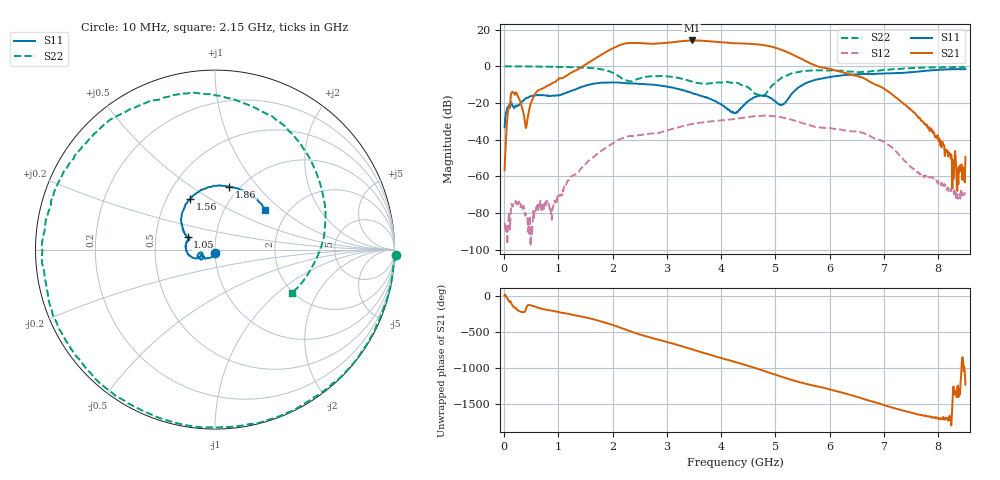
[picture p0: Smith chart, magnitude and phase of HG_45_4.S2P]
!Agilent Technologies,E5071C,MY46523237,B.13.01
!Date: Tue Sep 12 16:48:18 2023
!Data & Calibration Information:
!Freq	S11:SOLT2(ON)	S21:SOLT2(ON)	S12:SOLT2(ON)	S22:SOLT2(ON)
!PortZ  Port1:50+j0  Port2:50+j0
!Above PortZ is port z conversion or system Z0 setting when saving the data.
!When reading, reference impedance value at option line is always used.
# Hz S dB R 50
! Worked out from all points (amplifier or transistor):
!   850 points, 10 MHz to 8.5 GHz, reference 50 ohm
!   highest |S21| = 14.1 dB at 3.46 GHz (marker M1)
!   |S21| within 3 dB of that: 2.092 GHz to 4.878 GHz (2.786 GHz wide, 79.9 % of centre)
!   unconditionally stable (mu >= 1): 23.91 MHz to end of sweep
!   at 1.42 GHz: K = 40.33, MAG = 8.5 dB, |S12| = -55.8 dB
!   at 4.26 GHz: K = 2.85, MAG = 13.2 dB, |S12| = -28.6 dB
!   at 8.5 GHz: K = 14264.41, MAG = -34.9 dB, |S12| = -68.8 dB
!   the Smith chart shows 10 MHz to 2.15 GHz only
!   S11 on the Smith chart (normalised r, x): 10 MHz: 1.00, -0.04; 1.05 GHz: 0.73, +0.11; 1.56 GHz: 0.65, +0.41; 1.86 GHz: 0.90, +0.72; 2.15 GHz: 1.54, +0.78
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1e7  -33.31 -88.0  -56.67 11.4  -85.25 -36.6  0.08 -1.7
1.6e8  -21.73 -169.0  -14.35 -132.5  -76.61 76.8  -0.03 -30.6
1.05e9  -15.48 155.4  -6.52 130.0  -70.29 64.8  -0.35 -171.4
1.43e9  -11.14 131.2  -0.37 77.8  -55.26 35.7  -0.62 137.5
1.56e9  -10.07 116.6  2.14 55.5  -51.50 11.4  -0.84 118.3
1.86e9  -8.87 77.2  7.54 -5.7  -44.70 -49.0  -1.99 62.7
2.15e9  -8.97 38.1  11.77 -79.5  -39.62 -115.7  -6.18 -29.6
2.29e9  -9.22 19.4  12.72 -118.9  -38.15 -152.6  -8.02 -99.8
2.48e9  -9.52 -6.9  12.74 -167.7  -37.58 164.9  -6.78 176.7
2.84e9  -10.33 -64.5  12.50 115.9  -36.43 96.8  -5.39 88.3
3.14e9  -11.87 -114.3  13.30 53.8  -33.83 40.7  -5.98 26.8
3.46e9  -14.53 -159.6  14.13 -18.4  -31.49 -25.8  -8.27 -59.7
3.8e9  -17.75 159.2  13.66 -96.5  -30.08 -98.4  -9.36 -173.3
4.03e9  -21.34 121.9  13.03 -147.1  -29.39 -146.2  -8.69 125.6
4.26e9  -25.46 35.3  12.58 164.2  -28.61 167.4  -8.96 79.1
4.57e9  -17.67 -77.1  12.19 93.8  -27.40 99.0  -13.59 39.9
4.88e9  -16.69 -131.4  11.12 17.4  -27.01 24.2  -12.59 67.6
5.2e9  -19.11 -97.2  8.00 -62.4  -28.36 -54.2  -5.14 29.0
5.67e9  -7.94 -131.3  1.25 -159.7  -32.43 -150.9  -2.24 -51.0
6.34e9  -4.65 161.7  -3.97 74.8  -35.27 80.3  -2.83 -179.7
7.09e9  -3.78 86.8  -13.95 -97.7  -43.00 -100.8  -1.84 -25.0
8.5e9  -1.48 -105.0  -49.50 -153.6  -68.82 -26.5  -0.56 -169.5
